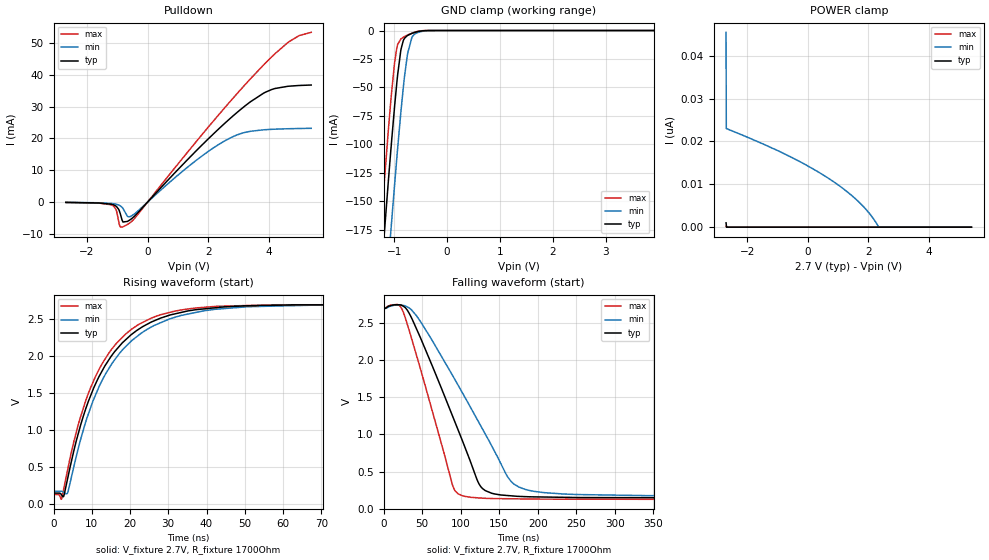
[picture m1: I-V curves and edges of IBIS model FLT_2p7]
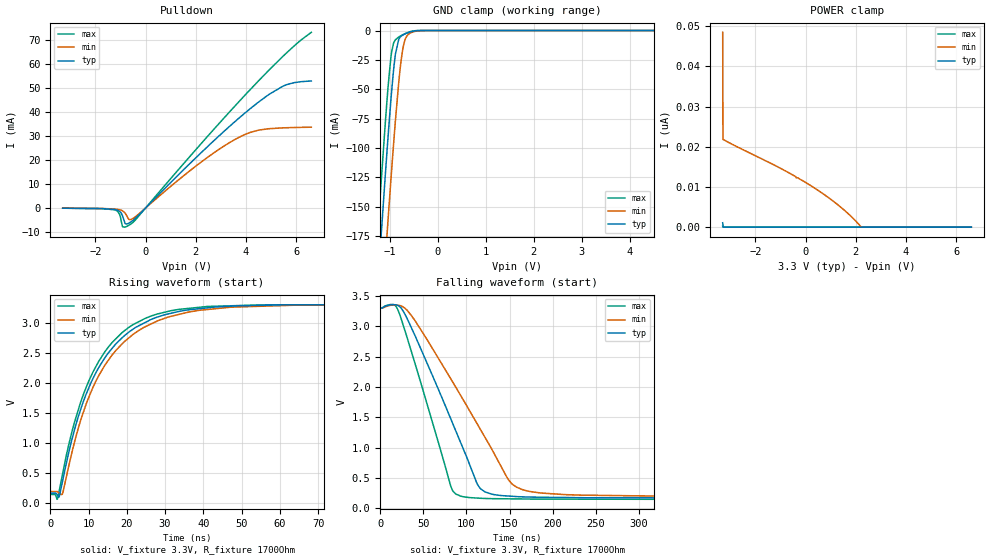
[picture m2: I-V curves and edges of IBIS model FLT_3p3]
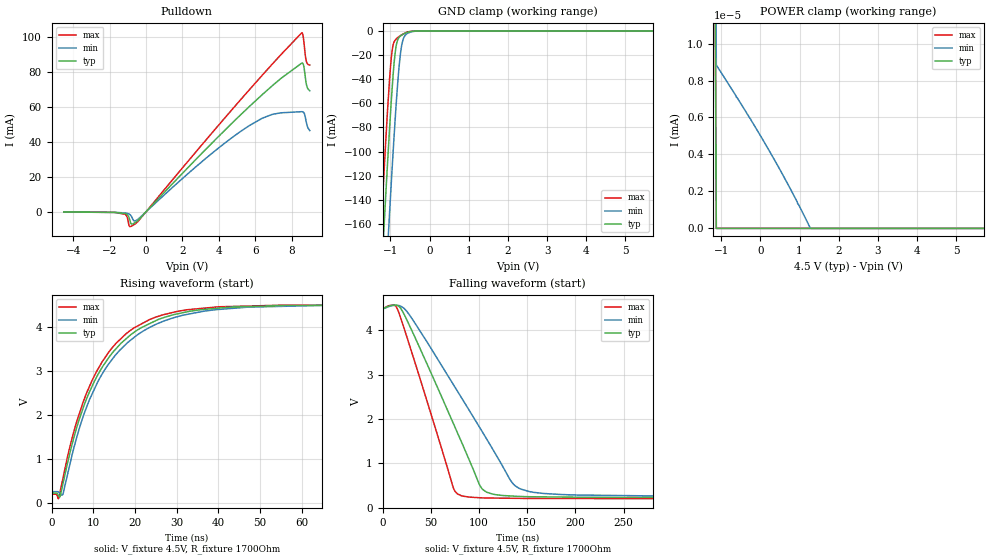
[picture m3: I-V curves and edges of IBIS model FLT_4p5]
|Texas Instruments Incorporated
|TPD2S300 USB Type C Short-to-VBUS and IEC ESD Protector for the CC Pins
| Device NAme#   Digital Voltage Range   Package-type   #pins
| TPD2S300WCSP   2.7V-4.5V   WCSP   9
[IBIS Ver]   4.1
[File name]   tpd2s300.ibs
[Date]   04/25/2017
[File Rev]   1.0
[Source]
| Texas Instruments Incorporated.
| Analog-eLab Design Center, HPA
| 12500 TI Blvd
| Dallas, TX -75243
[Notes]
| Rev 1.0: 04/25/2017
| - Initial version of the model
| - Model generated from simulations in SPECTRE
| - Model matched to SPICE simulation
| - C_comp although listed in numerical order of value are
|   obtained from varying PVT conditions. For PVT conditions for
|   each specific value refer the buffer description under
|   respective [Model]. IBIS model user is responsible for using
|   appropriate C_comp to simulate for Signal Integrity.
| - Non monotonic behavior result of buffer design
[Disclaimer]
| This model is designed as an aid for customers of Texas Instruments.
| TI and its licensors and suppliers make no warranties, either expressed
| or implied, with respect to this  model, including the warranties of
| merchantability or fitness for a particular purpose. The model is
| provided solely on an "as is" basis. The entire risk as to its quality
| and performance is with the customer.
[Copyright]
(C) Copyright 2017 Texas Instruments Incorporated.All rights reserved.
|   TPD2S300WCSP
[Component]   TPD2S300WCSP
[Manufacturer]  TI
[Package]   |9  WCSP
|   typ   min   max
R_pkg   0.005   0.005   0.005
L_pkg   0.20nH   0.2nH   0.2nH
C_pkg   0.6pF   0.6pF   0.6pF
[Pin]  signal_name model_name   R_pin   L_pin   C_pin
A1   C_CC1   NC   0.005   0.2nH   0.6pF
A2   VBIAS   power   0.005   0.2nH   0.6pF
A3   C_CC2   NC   0.005   0.2nH   0.6pF
B1   CC1   NC   0.005   0.2nH   0.6pF
B2   GND   gnd   0.005   0.2nH   0.6pF
B3   CC2   NC   0.005   0.2nH   0.6pF
C1   _FLT   FLT   0.005   0.2nH   0.6pF
C2   VPWR   power   0.005   0.2nH   0.6pF
C3   VM   VM   0.005   0.2nH   0.6pF
|   Model Selectors
[Model Selector] FLT
FLT_2p7   2.7V  digital Open_drain
FLT_3p3   3.3V  digital Open_drain
FLT_4p5   4.5V  digital Open_drain
[Model Selector] VM
vm_2p7   2.7V  digital Input
vm_3p3   3.3V  digital Input
vm_4p5   4.5V  digital Input
| Models and submodels in the file (6): FLT_2p7 (Open_drain), FLT_3p3 (Open_drain), FLT_4p5 (Open_drain), vm_2p7 (Input), vm_3p3 (Input), vm_4p5 (Input)
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|   FLT_2p7 Model
[Model]   FLT_2p7
Model_type   Open_drain
Polarity   Non-Inverting
Vmeas = 1.35
Vref = 2.7
Cref = 2pF
Rref = 1700
|   typ   min   max
C_comp   0.733905pF   0.632937pF   0.867242pF
|C_comp_pulldown   0.521106pF   0.49416pF   0.59162pF
| Where nom  PVT is Nominal Process, 2.7V, 27C
|   Fast PVT is Strong Process,  2.701V, -40C
|   Slow PVT is Weak Process,   2.699V, 125C
[Voltage Range]   2.7   2.699   2.701
[Temperature Range]   27   125   -40
[Pullup Reference]   2.7   2.699   2.701
[Pulldown Reference]   0   0   0
[Power Clamp Reference]   2.7   2.699   2.701
[GND Clamp Reference]   0   0   0
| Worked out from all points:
|   slope of the pulldown table from 0 to 0.405 V, typ, clamps not added: 96.9 ohm
|   GND clamp passes 1 mA (typ) near -0.56 V on its own axis
|   falling waveform, V_fixture 2.7V, R_fixture 1700Ohm: 20-80 % time 59.6ns typ, 81.8ns min, 41.9ns max; typ from 2.7 V to 0.145 V
|   rising waveform, V_fixture 2.7V, R_fixture 1700Ohm: 20-80 % time 13.1ns typ, 14ns min, 12.3ns max; typ from 0.145 V to 2.7 V
[Pulldown]
|   Voltage   I(typ)   I(min)   I(max)
-2.7V     -113uA     -96.19uA   -112.2uA
-1.21V    -657.5uA   -431.1uA   -846.1uA
-1.04V    -1.312mA   -679.4uA   -2.448mA
-901.8mV  -3.655mA   -1.189mA   -7.791mA
-812.7mV  -6.266mA   -2.007mA   -7.776mA
-626.4mV  -5.864mA   -4.645mA   -6.793mA
1.561V    15.68mA    12.78mA    18.48mA
2.735V    26.36mA    20.17mA    31.71mA
3.399V    31.54mA    22.24mA    38.77mA
4.096V    35.36mA    22.85mA    45.62mA
4.655V    36.39mA    23.04mA    50.3mA
5.4V      36.77mA    23.17mA    53.32mA
[GND Clamp]
|   Voltage   I(typ)   I(min)   I(max)
-2.7V     -1.153A    -1.222A    -1.111A
-1.258V   -221mA     -293.8mA   -175.3mA
-1.112V   -133mA     -205mA     -88.21mA
-1.064V   -105mA     -176.2mA   -61.46mA
-990.9mV  -65.36mA   -134.1mA   -27.33mA
-950.4mV  -45.54mA   -111.5mA   -15.1mA
-877.5mV  -18.03mA   -73.15mA   -7.573mA
-828.9mV  -8.862mA   -50.15mA   -5.912mA
-747.9mV  -4.304mA   -20.26mA   -3.93mA
-642.6mV  -2.136mA   -4.473mA   -1.936mA
-391.5mV  -58uA      -228.7uA   -21.68uA
5.4V      0A         0A         0A
[POWER Clamp]
|   Voltage   I(typ)   I(min)   I(max)
-2.7V     1.011nA    45.48nA    206.1pA
-2.692V   505.7pA    23.02nA    103.1pA
-2.684V   0A         23nA       0A
-942.3mV  0A         17.7nA     0A
-140.4mV  0A         14.84nA    0A
685.8mV   0A         11.38nA    0A
1.269V    0A         8.425nA    0A
1.731V    0A         5.554nA    0A
2.079V    0A         2.773nA    0A
2.338V    0A         23.14pA    0A
5.4V      0A         0A         0A
[Ramp]
R_load = 1700
|   typ   min   max
dV/dt_r   1.53308/1.31057e-08   1.51731/1.3962e-08   1.54522/1.22413e-08
dV/dt_f   1.53308/5.95095e-08   1.51731/8.16584e-08   1.54522/4.18818e-08
[Falling Waveform]
V_fixture = 2.7V
V_fixture_min = 2.699V
V_fixture_max = 2.701V
R_fixture = 1700Ohm
C_fixture = 0F
|   Time   V(typ)   V(min)   V(max)
0s        2.7V       2.699V     2.701V
23.92ns   2.735V     2.737V     2.682V
42.3ns    2.427V     2.6V       2.075V
89.88ns   1.235V     1.785V     302.9mV
104.5ns   853.6mV    1.517V     167.5mV
122.5ns   359.4mV    1.181V     145.5mV
131.8ns   243.8mV    1.007V     139.5mV
165.5ns   172.9mV    365.9mV    133.1mV
195.4ns   158.6mV    232.8mV    129.4mV
1us       144.9mV    170.1mV    125.6mV
[Rising Waveform]
V_fixture = 2.7V
V_fixture_min = 2.699V
V_fixture_max = 2.701V
R_fixture = 1700Ohm
C_fixture = 0F
|   Time   V(typ)   V(min)   V(max)
0s        144.9mV    170.1mV    125.6mV
2.095ns   122.2mV    169.9mV    63.69mV
2.654ns   101.6mV    154.2mV    198.7mV
3.674ns   337.7mV    146.5mV    456.4mV
6.231ns   906.3mV    702mV      1.028V
8.987ns   1.37V      1.199V     1.479V
16.25ns   2.079V     1.97V      2.163V
26.19ns   2.477V     2.414V     2.529V
42.55ns   2.658V     2.637V     2.676V
1us       2.7V       2.699V     2.701V
|   FLT_3p3 Model
[Model]   FLT_3p3
Model_type   Open_drain
Polarity   Non-Inverting
Vmeas = 1.65
Vref = 3.3
Cref = 2pF
Rref = 1700
|   typ   min   max
C_comp   0.723726pF   0.622931pF   0.849555pF
|C_comp_pulldown   0.504243pF   0.472759pF   0.574963pF
| Where nom  PVT is Nominal Process, 3.3V, 27C
|   Fast PVT is Strong Process,  3.301V, -40C
|   Slow PVT is Weak Process,   3.299V, 125C
[Voltage Range]   3.3   3.299   3.301
[Temperature Range]   27   125   -40
[Pullup Reference]   3.3   3.299   3.301
[Pulldown Reference]   -0   0   -0
[Power Clamp Reference]   3.3   3.299   3.301
[GND Clamp Reference]   0   0   0
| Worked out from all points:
|   slope of the pulldown table from 0 to 0.495 V, typ, clamps not added: 93.6 ohm
|   GND clamp passes 1 mA (typ) near -0.56 V on its own axis
|   falling waveform, V_fixture 3.3V, R_fixture 1700Ohm: 20-80 % time 56ns typ, 76.8ns min, 39.4ns max; typ from 3.3 V to 0.172 V
|   rising waveform, V_fixture 3.3V, R_fixture 1700Ohm: 20-80 % time 12.9ns typ, 13.7ns min, 12ns max; typ from 0.172 V to 3.3 V
[Pulldown]
|   Voltage   I(typ)   I(min)   I(max)
-3.3V     -88.02uA   -77.83uA   -85.47uA
-1.261V   -592.4uA   -412.5uA   -719.1uA
-1.033V   -1.419mA   -738.4uA   -2.691mA
-914.1mV  -3.408mA   -1.188mA   -7.824mA
-815.1mV  -6.475mA   -2.095mA   -7.993mA
-676.5mV  -6.353mA   -4.61mA    -7.274mA
-577.5mV  -5.749mA   -4.791mA   -6.616mA
2.135V    22.28mA    18.53mA    25.92mA
3.759V    37.84mA    29.67mA    44.8mA
4.501V    44.2mA     32.47mA    53.06mA
5.471V    50.81mA    33.42mA    63.26mA
6.6V      52.98mA    33.69mA    73.26mA
[GND Clamp]
|   Voltage   I(typ)   I(min)   I(max)
-3.3V     -1.548A    -1.616A    -1.507A
-1.261V   -222.5mA   -295.3mA   -176.8mA
-1.181V   -174.1mA   -246.7mA   -128.6mA
-1.063V   -104.3mA   -175.5mA   -60.82mA
-1.043V   -93.19mA   -163.9mA   -50.63mA
-973.5mV  -56.59mA   -124.3mA   -21.25mA
-884.4mV  -19.98mA   -76.61mA   -7.885mA
-815.1mV  -7.5mA     -44.17mA   -5.526mA
-755.7mV  -4.531mA   -22.51mA   -4.098mA
-646.8mV  -2.203mA   -4.715mA   -2.006mA
-260.7mV  -1.974uA   -17.88uA   -404.4nA
6.6V      0A         0A         0A
[POWER Clamp]
|   Voltage   I(typ)   I(min)   I(max)
-3.3V     1.094nA    48.44nA    248pA
-3.29V    547.2pA    21.82nA    124pA
-3.28V    0A         21.79nA    0A
-1.003V   0A         14.65nA    0A
293.7mV   0A         9.981nA    0A
917.4mV   0A         7.321nA    0A
1.412V    0A         4.909nA    0A
1.818V    0A         2.642nA    0A
2.214V    0A         41.76pA    0A
6.6V      0A         0A         0A
[Ramp]
R_load = 1700
|   typ   min   max
dV/dt_r   1.87706/1.29034e-08   1.86037/1.37072e-08   1.89043/1.20385e-08
dV/dt_f   1.87706/5.59552e-08   1.86038/7.67951e-08   1.89043/3.9388e-08
[Falling Waveform]
V_fixture = 3.3V
V_fixture_min = 3.299V
V_fixture_max = 3.301V
R_fixture = 1700Ohm
C_fixture = 0F
|   Time   V(typ)   V(min)   V(max)
0s        3.3V       3.299V     3.301V
20.42ns   3.343V     3.345V     3.271V
36.33ns   2.967V     3.171V     2.571V
82.2ns    1.461V     2.125V     351.3mV
95.87ns   996mV      1.798V     194.1mV
112.6ns   404.1mV    1.39V      171mV
121.5ns   272.9mV    1.171V     164.6mV
151.6ns   201.5mV    422mV      158.2mV
185.8ns   185mV      254.8mV    153.4mV
1us       171.6mV    198.3mV    150.3mV
[Rising Waveform]
V_fixture = 3.3V
V_fixture_min = 3.299V
V_fixture_max = 3.301V
R_fixture = 1700Ohm
C_fixture = 0F
|   Time   V(typ)   V(min)   V(max)
0s        171.6mV    198.3mV    150.3mV
1.869ns   138.9mV    197mV      72.27mV
2.323ns   110.7mV    174mV      208.9mV
3.17ns    358.5mV    158.3mV    477mV
5.704ns   1.074V     859.6mV    1.201V
8.929ns   1.74V      1.565V     1.854V
16.24ns   2.58V      2.47V      2.676V
24.54ns   2.994V     2.924V     3.062V
41.08ns   3.246V     3.218V     3.269V
1us       3.3V       3.299V     3.301V
|   FLT_4p5 Model
[Model]   FLT_4p5
Model_type   Open_drain
Polarity   Non-Inverting
Vmeas = 2.25
Vref = 4.5
Cref = 2pF
Rref = 1700
|   typ   min   max
C_comp   0.703692pF   0.607712pF   0.81883pF
|C_comp_pulldown   0.479244pF   0.443812pF   0.550457pF
| Where nom  PVT is Nominal Process, 4.5V, 27C
|   Fast PVT is Strong Process,  4.501V, -40C
|   Slow PVT is Weak Process,   4.499V, 125C
[Voltage Range]   4.5   4.499   4.501
[Temperature Range]   27   125   -40
[Pullup Reference]   4.5   4.499   4.501
[Pulldown Reference]   0   0   0
[Power Clamp Reference]   4.5   4.499   4.501
[GND Clamp Reference]   0   0   0
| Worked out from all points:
|   slope of the pulldown table from 0 to 0.675 V, typ, clamps not added: 90.1 ohm
|   GND clamp passes 1 mA (typ) near -0.56 V on its own axis
|   POWER clamp passes 1 mA (typ) near -4.14 V on its own axis
|   falling waveform, V_fixture 4.5V, R_fixture 1700Ohm: 20-80 % time 52ns typ, 71.4ns min, 36.7ns max; typ from 4.5 V to 0.226 V
|   rising waveform, V_fixture 4.5V, R_fixture 1700Ohm: 20-80 % time 12.6ns typ, 13.3ns min, 11.8ns max; typ from 0.226 V to 4.5 V
[Pulldown]
|   Voltage   I(typ)   I(min)   I(max)
-4.5V     -61.25uA   -56.69uA   -58.03uA
-1.125V   -962.6uA   -605.7uA   -1.369mA
-895.5mV  -4.217mA   -1.401mA   -8.316mA
-706.5mV  -6.77mA    -4.445mA   -7.655mA
-409.5mV  -4.515mA   -3.917mA   -5.145mA
3.155V    34.38mA    29.43mA    39.35mA
5.652V    59.97mA    49.15mA    69.5mA
6.934V    72.09mA    55.76mA    84.45mA
8.555V    85.04mA    57.31mA    102.4mA
8.676V    83.01mA    56.72mA    97.17mA
8.811V    73.09mA    51.19mA    86.06mA
9V        69.24mA    46.5mA     83.99mA
[GND Clamp]
|   Voltage   I(typ)   I(min)   I(max)
-4.5V     -2.341A    -2.406A    -2.301A
-1.26V    -222.1mA   -294.9mA   -176.4mA
-1.125V   -140.4mA   -212.6mA   -95.42mA
-1.071V   -109.1mA   -180.4mA   -65.29mA
-1.017V   -79.09mA   -149mA     -38.28mA
-963mV    -51.47mA   -118.5mA   -18.17mA
-909mV    -28.2mA    -89.28mA   -9.382mA
-855mV    -12.81mA   -62.17mA   -6.724mA
-733.5mV  -3.924mA   -16.54mA   -3.629mA
-666mV    -2.526mA   -6.091mA   -2.337mA
-585mV    -1.327mA   -2.388mA   -1.081mA
9V        0A         0A         0A
[POWER Clamp]
|   Voltage   I(typ)   I(min)   I(max)
-4.5V     41.94mA    30.54mA    50.37mA
-3.96V    1.327uA    1.473uA    1.248uA
-1.125V   0A         8.841nA    0A
-625.5mV  0A         7.179nA    0A
-612mV    0A         7.092nA    0A
-598.5mV  0A         7.089nA    0A
-247.5mV  0A         5.909nA    0A
265.5mV   0A         4.055nA    0A
765mV     0A         2.141nA    0A
1.278V    0A         0A         0A
9V        0A         0A         0A
[Ramp]
R_load = 1700
|   typ   min   max
dV/dt_r   2.56443/1.25729e-08   2.54574/1.33435e-08   2.58043/1.17397e-08
dV/dt_f   2.56443/5.19934e-08   2.54574/7.13469e-08   2.58043/3.67068e-08
[Falling Waveform]
V_fixture = 4.5V
V_fixture_min = 4.499V
V_fixture_max = 4.501V
R_fixture = 1700Ohm
C_fixture = 0F
|   Time   V(typ)   V(min)   V(max)
0s        4.5V       4.499V     4.501V
16.16ns   4.551V     4.561V     4.444V
29.08ns   4.055V     4.312V     3.588V
73.3ns    1.906V     2.782V     458.3mV
83.41ns   1.406V     2.426V     258.1mV
100.9ns   501.7mV    1.802V     221.1mV
108.2ns   346.1mV    1.541V     216mV
136.5ns   257.3mV    512.9mV    209.1mV
167.3ns   241.4mV    317.8mV    204.3mV
1us       226mV      256mV      200.3mV
[Rising Waveform]
V_fixture = 4.5V
V_fixture_min = 4.499V
V_fixture_max = 4.501V
R_fixture = 1700Ohm
C_fixture = 0F
|   Time   V(typ)   V(min)   V(max)
0s        226mV      256mV      200.3mV
1.649ns   163.6mV    245.2mV    98.74mV
2.625ns   402.5mV    185.3mV    527.6mV
5.521ns   1.553V     1.324V     1.694V
8.01ns    2.279V     2.087V     2.41V
11.1ns    2.919V     2.762V     3.042V
15.42ns   3.504V     3.374V     3.627V
25.11ns   4.15V      4.066V     4.229V
39.99ns   4.428V     4.398V     4.458V
1us       4.5V       4.499V     4.501V
